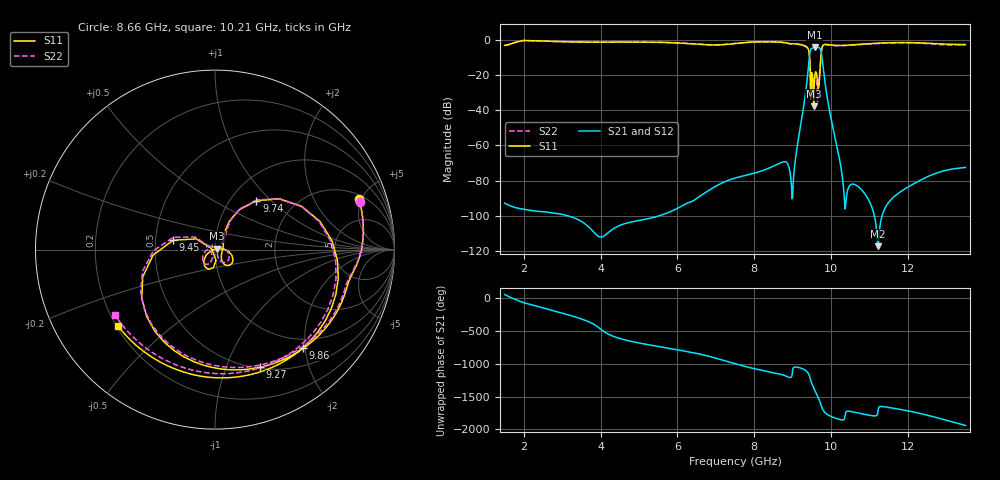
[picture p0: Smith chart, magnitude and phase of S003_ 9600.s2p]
# Hz S DB R 50
! Planar, S50180, , 20.4.1/1
! Date: 14.12.2021 18:52:41
! Data: Format (Calibration Info)
! Freq	S11:dB/Ang(--)	S21:dB/Ang(--)	S12:dB/Ang(--)	S22:dB/Ang(--)
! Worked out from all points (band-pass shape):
!   1201 points, 1.5 GHz to 13.5 GHz, reference 50 ohm
!   highest |S21| = -4.26 dB at 9.58 GHz (marker M1); lowest = -117.3 dB at 11.22 GHz (marker M2)
!   |S21| within 3 dB of the highest: 9.452 GHz to 9.745 GHz (292.9 MHz wide, 3.05 % of centre)
!   lowest |S11| = -37.8 dB at 9.55 GHz (marker M3), VSWR 1.03, Z = 51.1 + j0.625 ohm
!   |S11| at or under -10 dB: 9.442 GHz to 9.736 GHz (293.7 MHz wide, 3.06 % of centre)
!   |S22| runs from -35.2 to -0.4 dB; largest |S21 - S12| = 2.2e-06
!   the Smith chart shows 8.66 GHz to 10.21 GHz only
!   S11 on the Smith chart (normalised r, x): 8.66 GHz: 2.36, +4.78; 9.27 GHz: 0.51, -1.32; 9.45 GHz: 0.62, +0.07; 9.74 GHz: 1.31, +0.82; 9.86 GHz: 0.83, -1.96; 10.21 GHz: 0.21, -0.33
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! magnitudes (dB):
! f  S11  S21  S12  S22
! 1.5 GHz  -3.2  -92.8  -92.8  -3.3
! 3.5 GHz  -1.3  -103.2  -103.2  -1.3
! 5.5 GHz  -1.5  -100.2  -100.2  -1.5
! 7.5 GHz  -2.1  -78.6  -78.6  -2.1
! 8.66 GHz  -1.4  -70.2  -70.2  -1.4
! 8.83 GHz  -1.8  -69.5  -69.5  -1.9
! 9 GHz  -2.3  -88.6  -88.6  -2.4
! 9.27 GHz  -3.1  -40.5  -40.5  -3.3
! 9.38 GHz  -4.3  -22.4  -22.4  -4.6
! 9.45 GHz  -12.4  -7.6  -7.6  -12.3
! 9.5 GHz  -18.7  -5.0  -5.0  -20.2
! 9.55 GHz  -37.8  -4.4  -4.4  -33.3
! 9.58 GHz  -20.0  -4.3  -4.3  -21.5
! 9.67 GHz  -27.7  -4.4  -4.4  -26.8
! 9.74 GHz  -8.9  -6.6  -6.6  -8.8
! 9.79 GHz  -3.3  -14.6  -14.6  -3.4
! 9.86 GHz  -2.7  -26.8  -26.8  -2.9
! 10.21 GHz  -3.2  -66.6  -66.6  -3.5
! 10.36 GHz  -3.2  -94.7  -94.7  -3.4
! 11.22 GHz  -2.0  -117.3  -117.3  -2.2
! 11.5 GHz  -1.7  -92.4  -92.4  -1.9
! 13.5 GHz  -2.8  -72.6  -72.6  -2.8
